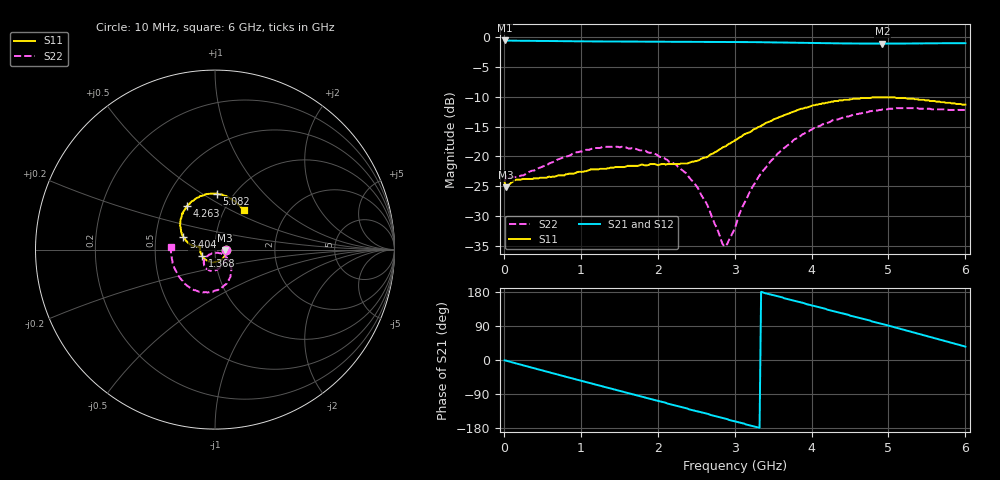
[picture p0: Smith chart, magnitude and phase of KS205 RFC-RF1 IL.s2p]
!Agilent	"Technologies,E5071B,JP1KK00126,A.08.11"
!Date:	Wed	Mar	27	12:09:31	2013
!Data	&	Calibration	Information:
!Freq	S11:SOLT2(ON)	S21:SOLT2(ON)	S12:SOLT2(ON)	S22:SOLT2(ON)
#	Hz	S	dB	R	50
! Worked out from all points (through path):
!   301 points, 10 MHz to 6 GHz, reference 50 ohm
!   highest |S21| = -0.52 dB at 10 MHz (marker M1); lowest = -1.1 dB at 4.922 GHz (marker M2)
!   group delay of S21, straight-line fit = 150 ps
!   lowest |S11| = -25.2 dB at 29.97 MHz (marker M3), VSWR 1.12, Z = 55.8 - j0.245 ohm
!   |S11| at or under -10 dB: start of sweep to end of sweep
!   |S22| runs from -35.1 to -11.9 dB; largest |S21 - S12| = 0.016
!   S11 on the Smith chart (normalised r, x): 10 MHz: 1.13, -0.00; 1.368 GHz: 0.86, -0.06; 3.404 GHz: 0.69, +0.10; 4.263 GHz: 0.66, +0.35; 5.082 GHz: 0.84, +0.58; 6 GHz: 1.23, +0.58
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1e7  -24.40 -1.3  -0.52 -1.0  -0.52 -1.0  -24.40 -0.5
2.996667e7  -25.20 -2.3  -0.54 -1.7  -0.54 -1.8  -23.30 -0.7
1.697333e8  -23.90 -18.4  -0.57 -9.6  -0.57 -9.6  -23.50 -15.6
5.091667e8  -23.60 -59.1  -0.60 -28.0  -0.60 -28.1  -21.70 -47.0
1.0283e9  -22.60 -123.0  -0.67 -56.0  -0.67 -56.0  -19.10 -82.5
1.367733e9  -22.00 -154.0  -0.70 -74.1  -0.70 -74.1  -18.40 -99.0
1.707167e9  -21.60 -177.0  -0.72 -92.1  -0.72 -92.2  -18.70 -113.0
2.006667e9  -21.50 171.0  -0.74 -108.0  -0.74 -108.0  -19.90 -127.0
2.246267e9  -21.30 167.0  -0.74 -121.0  -0.74 -121.0  -21.50 -136.0
2.505833e9  -20.80 169.0  -0.75 -135.0  -0.75 -135.0  -25.00 -140.0
2.865233e9  -18.40 171.0  -0.76 -154.0  -0.76 -154.0  -35.10 -91.6
3.005e9  -17.30 169.0  -0.78 -162.0  -0.78 -162.0  -32.00 -44.4
3.1847e9  -16.00 165.0  -0.80 -172.0  -0.80 -172.0  -26.30 -32.6
3.404333e9  -14.40 158.0  -0.83 176.0  -0.83 176.0  -21.90 -34.1
3.604e9  -13.30 151.0  -0.87 166.0  -0.87 165.0  -19.00 -42.1
4.0233e9  -11.40 133.0  -0.96 143.0  -0.96 143.0  -15.30 -59.7
4.2629e9  -10.80 123.0  -1.00 130.0  -1.00 130.0  -14.00 -71.0
4.9218e9  -10.10 94.3  -1.06 95.0  -1.06 95.0  -12.10 -106.0
5.001667e9  -10.10 90.9  -1.05 90.7  -1.05 90.7  -12.00 -111.0
5.081533e9  -10.10 87.7  -1.05 86.4  -1.05 86.5  -12.00 -116.0
5.5208e9  -10.60 70.6  -1.00 62.3  -1.00 62.4  -12.00 -145.0
6e9  -11.30 54.0  -0.98 35.3  -0.98 35.4  -12.20 177.0
